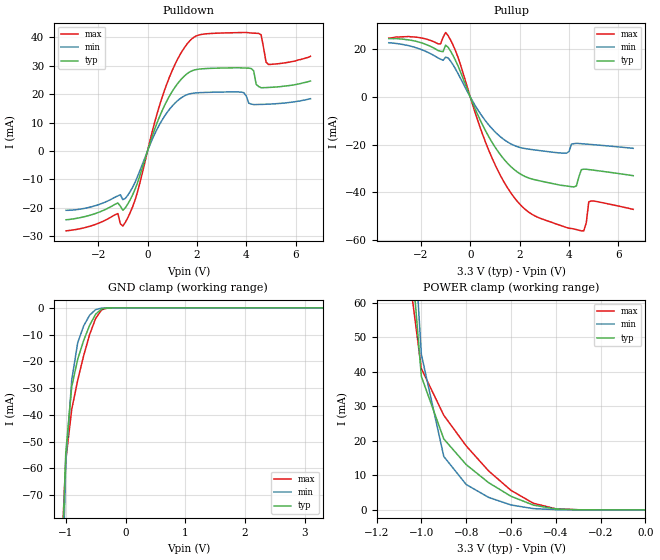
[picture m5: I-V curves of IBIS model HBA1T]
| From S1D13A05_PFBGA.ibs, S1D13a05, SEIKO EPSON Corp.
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[Model]   HBA1T
Model_type I/O
Enable Active-Low
Polarity Non-Inverting
Vinh=2.0
Vinl=0.8
C_comp   5p   4p   6p
[Temperature Range] 50   100   0
[Voltage Range]   3.3   3.0   3.6
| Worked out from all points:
|   slope of the pulldown table from 0 to 0.495 V, typ, clamps not added: 40.4 ohm
|   slope of the pullup table from 0 to 0.495 V, typ, clamps not added: 42.4 ohm
|   GND clamp passes 1 mA (typ) near -0.43 V on its own axis
|   POWER clamp passes 1 mA (typ) near -0.47 V on its own axis
[Pullup]
-3.3V     24.48mA    22.74mA    24.65mA
-1.2V     19.16mA    15.83mA    22.29mA
-900mV    20.89mA    16.4mA     25.77mA
1V        -20.97mA   -14.6mA    -28.3mA
1.7V      -29.74mA   -19.97mA   -41.07mA
2.4V      -34.12mA   -21.95mA   -48.56mA
3.9V      -37.33mA   -23.58mA   -54.78mA
4.2V      -37.75mA   -19.6mA    -55.39mA
4.5V      -30.52mA   -19.62mA   -56.18mA
4.7V      -30.33mA   -19.79mA   -52.72mA
4.8V      -30.46mA   -19.87mA   -43.99mA
6.6V      -33.02mA   -21.56mA   -47.15mA
[Pulldown]
-3.3V     -24.24mA   -20.91mA   -28.16mA
-1.2V     -18.34mA   -15.83mA   -22.07mA
-1.1V     -19.46mA   -15.42mA   -25.67mA
-900mV    -20.04mA   -16.72mA   -25.18mA
-400mV    -11.05mA   -8.882mA   -14.26mA
800mV     17.95mA    13.68mA    24.09mA
1.9V      28.56mA    20.41mA    40.22mA
3.8V      29.29mA    20.75mA    41.74mA
4.2V      29.07mA    16.54mA    41.59mA
4.5V      22.72mA    16.39mA    41.43mA
4.9V      22.39mA    16.51mA    30.48mA
6.6V      24.66mA    18.42mA    33.38mA
[GND Clamp]
-3.3V     -3.904A    -3.557A    -4.353A
-1.1V     -118.9mA   -145mA     -106mA
-1V       -54.09mA   -58.05mA   -56.96mA
-900mV    -29.42mA   -26.86mA   -37.89mA
-800mV    -19.16mA   -13.01mA   -27.02mA
-700mV    -12.15mA   -6.718mA   -17.78mA
-600mV    -6.477mA   -2.726mA   -9.93mA
-500mV    -2.365mA   -667.1uA   -3.94mA
-400mV    -431.6uA   -96.18uA   -746.4uA
-300mV    -40.31uA   -9.839uA   -57.18uA
3.3V      5.041nA    4.639uA    977pA
[POWER Clamp]
-3.3V     3.948A     3.603A     4.377A
-1.1V     117.5mA    151.4mA    91.09mA
-1V       38.6mA     44.98mA    40.87mA
-900mV    20.53mA    15.46mA    27.37mA
-800mV    13.1mA     7.338mA    18.51mA
-700mV    7.867mA    3.611mA    11.28mA
-600mV    3.929mA    1.414mA    5.638mA
-500mV    1.368mA    349.4uA    1.9mA
-400mV    257.4uA    50.44uA    302.5uA
-300mV    26.21uA    4.639uA    23.79uA
0V        5.041nA    5.145nA    1.201nA
[Ramp]
R_load=50
dV/dt_r   9.131E-1/3.201E-10   6.301E-1/3.899E-10   1.193E+0/2.612E-10
dV/dt_f   8.550E-1/4.265E-10   6.142E-1/4.874E-10   1.155E+0/3.440E-10
